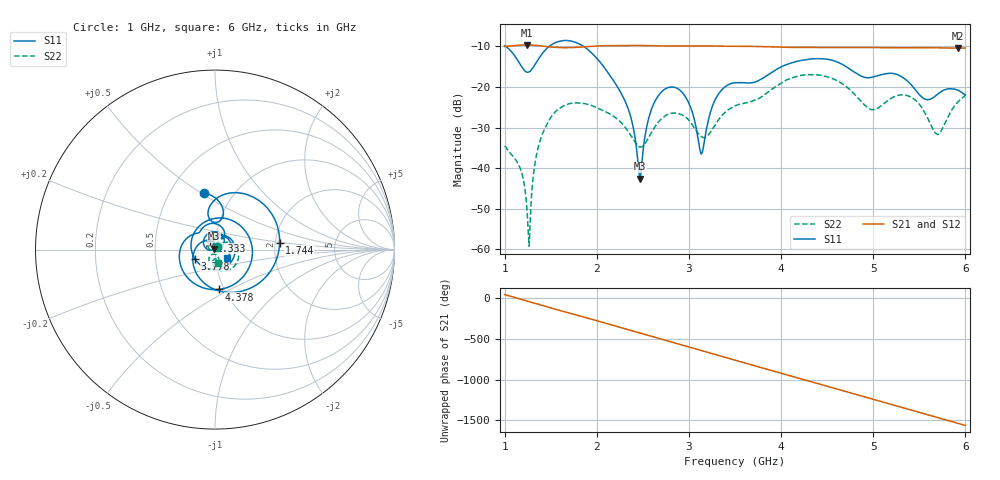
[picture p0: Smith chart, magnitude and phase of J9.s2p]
!Agilent Technologies,E8364B,MY43040528,A.07.50.67
!Agilent E8364B: A.07.50.67
!Date: Sunday, March 01, 2026 15:29:45
!Correction: S11(Full 2 Port(1,2))
!S21(Full 2 Port(1,2))
!S12(Full 2 Port(1,2))
!S22(Full 2 Port(1,2))
!S2P File: Measurements: S11, S21, S12, S22:
# Hz S  dB  R 50
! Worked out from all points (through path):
!   451 points, 1 GHz to 6 GHz, reference 50 ohm
!   highest |S21| = -9.66 dB at 1.244 GHz (marker M1); lowest = -10.4 dB at 5.922 GHz (marker M2)
!   group delay of S21, straight-line fit = 892 ps
!   lowest |S11| = -42.6 dB at 2.467 GHz (marker M3), VSWR 1.01, Z = 49.5 + j0.525 ohm
!   |S11| at or under -10 dB: 1.011 GHz to 1.485 GHz (474.5 MHz wide, 38 % of centre); 1.856 GHz to end of sweep
!   |S22| runs from -59.2 to -17.0 dB; largest |S21 - S12| = 0.0015
!   S11 on the Smith chart (normalised r, x): 1 GHz: 0.73, +0.51; 1.744 GHz: 2.11, +0.18; 2.333 GHz: 0.94, +0.10; 3.778 GHz: 0.79, -0.08; 4.378 GHz: 0.94, -0.44; 6 GHz: 1.14, -0.10
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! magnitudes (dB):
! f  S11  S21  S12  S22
! 1 GHz  -9.8  -10.0  -10.1  -34.5
! 1.178 GHz  -14.8  -9.7  -9.7  -40.6
! 1.244 GHz  -16.4  -9.7  -9.7  -50.5
! 1.278 GHz  -16.1  -9.7  -9.7  -52.9
! 1.422 GHz  -11.4  -10.0  -10.0  -31.0
! 1.744 GHz  -8.8  -10.3  -10.3  -24.0
! 1.844 GHz  -9.8  -10.2  -10.2  -24.0
! 2.333 GHz  -24.9  -9.8  -9.8  -30.7
! 2.467 GHz  -42.6  -9.8  -9.8  -34.8
! 2.667 GHz  -22.2  -9.9  -9.9  -28.7
! 2.933 GHz  -21.5  -9.9  -9.9  -27.0
! 3.133 GHz  -36.5  -9.9  -9.9  -32.2
! 3.289 GHz  -23.0  -9.9  -10.0  -29.2
! 3.5 GHz  -19.0  -10.0  -10.0  -24.7
! 3.778 GHz  -18.2  -10.1  -10.1  -22.6
! 4.344 GHz  -13.1  -10.3  -10.3  -17.0
! 4.378 GHz  -13.0  -10.3  -10.3  -17.0
! 5.167 GHz  -16.7  -10.4  -10.4  -23.2
! 5.433 GHz  -20.0  -10.3  -10.4  -22.8
! 5.7 GHz  -21.8  -10.4  -10.4  -31.7
! 5.922 GHz  -20.8  -10.4  -10.5  -23.6
! 6 GHz  -22.0  -10.4  -10.5  -22.1
